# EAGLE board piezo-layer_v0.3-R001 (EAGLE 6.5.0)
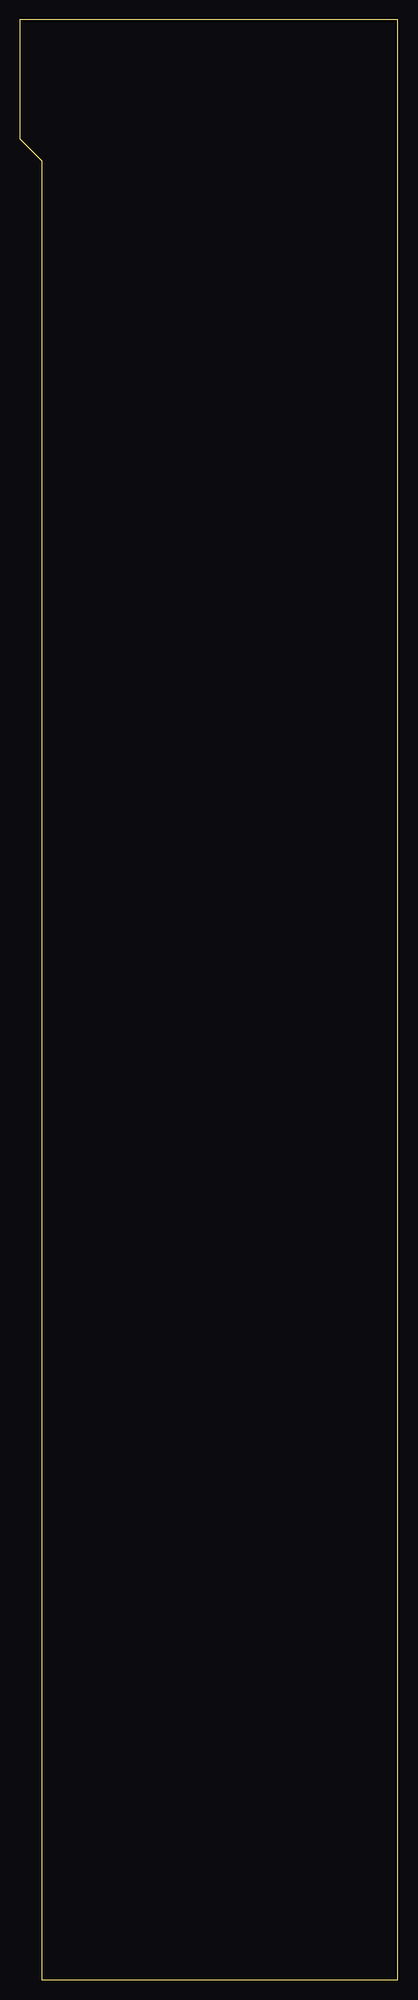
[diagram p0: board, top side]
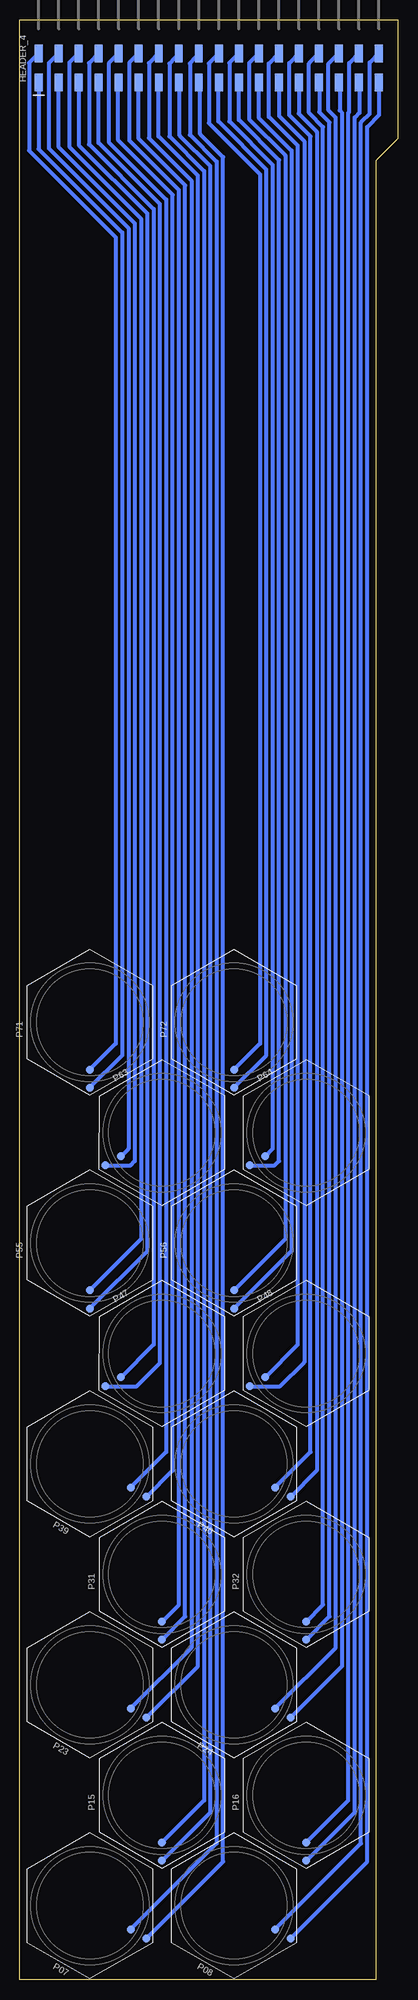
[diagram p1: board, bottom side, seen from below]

Size 48 x 248.5 mm. Coordinates in mm from the lower left corner, seen from the top.
Outline: 2.8,0 48,0 48,248.5 0,248.5 0,233.4 2.8,230.6 2.8,0
Copper layers (1*16): Top 0.009mm / dielectric 0.2mm / Bottom 0.018mm
Design rules "1L-0.2-0.15_0.3mm *": minimum track width 0.2mm, minimum drill 0.3mm, track to track 0.15mm, track to pad 0.15mm, pad to pad 0.15mm, via to via 0.15mm, smd to smd 0.15mm, copper to edge 0.5mm, drill to drill 1mm, minimum pad ring 10mil, minimum via ring 8mil, stop-mask expansion 4mil, vias tented up to drill 0mil, thermal gap 10mil

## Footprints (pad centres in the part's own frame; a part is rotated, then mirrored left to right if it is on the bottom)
2X18_2.54_90_SMD = smd 1 x 2.2: 1 -21.59,-1.84; 2 -21.59,1.84; 3 -19.05,-1.84; 4 -19.05,1.84; 5 -16.51,-1.84; 6 -16.51,1.84; 7 -13.97,-1.84; 8 -13.97,1.84; 9 -11.43,-1.84; 10 -11.43,1.84; 11 -8.89,-1.84; 12 -8.89,1.84; 13 -6.35,-1.84; 14 -6.35,1.84; 15 -3.81,-1.84; 16 -3.81,1.84; 17 -1.27,-1.84; 18 -1.27,1.84; 19 1.27,-1.84; 20 1.27,1.84; 21 3.81,-1.84; 22 3.81,1.84; 23 6.35,-1.84; 24 6.35,1.84; 25 8.89,-1.84; 26 8.89,1.84; 27 11.43,-1.84; 28 11.43,1.84; 29 13.97,-1.84; 30 13.97,1.84; 31 16.51,-1.84; 32 16.51,1.84; 33 19.05,-1.84; 34 19.05,1.84; 35 21.59,-1.84; 36 21.59,1.84
PIEZO-BENDER-HEX_16MM_1+_1- = smd 1 x 1: PAD1 -8.3,0; TIP1 -6,0

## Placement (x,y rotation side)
HEADER_4  HEADER_2X18-2.54_90_SMD  [2X18_2.54_90_SMD]  24,242.4 0 bottom
P07  PIEZO-BENDER-HEX_1-1  [PIEZO-BENDER-HEX_16MM_1+_1-]  39.1,9.4 150 bottom
P08  PIEZO-BENDER-HEX_1-1  [PIEZO-BENDER-HEX_16MM_1+_1-]  20.8,9.4 150 bottom
P15  PIEZO-BENDER-HEX_1-1  [PIEZO-BENDER-HEX_16MM_1+_1-]  29.95,23.4 90 bottom
P16  PIEZO-BENDER-HEX_1-1  [PIEZO-BENDER-HEX_16MM_1+_1-]  11.65,23.4 90 bottom
P23  PIEZO-BENDER-HEX_1-1  [PIEZO-BENDER-HEX_16MM_1+_1-]  39.1,37.4 150 bottom
P24  PIEZO-BENDER-HEX_1-1  [PIEZO-BENDER-HEX_16MM_1+_1-]  20.8,37.4 150 bottom
P31  PIEZO-BENDER-HEX_1-1  [PIEZO-BENDER-HEX_16MM_1+_1-]  29.95,51.4 90 bottom
P32  PIEZO-BENDER-HEX_1-1  [PIEZO-BENDER-HEX_16MM_1+_1-]  11.65,51.4 90 bottom
P39  PIEZO-BENDER-HEX_1-1  [PIEZO-BENDER-HEX_16MM_1+_1-]  39.1,65.4 150 bottom
P40  PIEZO-BENDER-HEX_1-1  [PIEZO-BENDER-HEX_16MM_1+_1-]  20.8,65.4 150 bottom
P47  PIEZO-BENDER-HEX_1-1  [PIEZO-BENDER-HEX_16MM_1+_1-]  29.95,79.4 30 bottom
P48  PIEZO-BENDER-HEX_1-1  [PIEZO-BENDER-HEX_16MM_1+_1-]  11.65,79.4 30 bottom
P55  PIEZO-BENDER-HEX_1-1  [PIEZO-BENDER-HEX_16MM_1+_1-]  39.1,93.4 90 bottom
P56  PIEZO-BENDER-HEX_1-1  [PIEZO-BENDER-HEX_16MM_1+_1-]  20.8,93.4 90 bottom
P63  PIEZO-BENDER-HEX_1-1  [PIEZO-BENDER-HEX_16MM_1+_1-]  29.95,107.4 30 bottom
P64  PIEZO-BENDER-HEX_1-1  [PIEZO-BENDER-HEX_16MM_1+_1-]  11.65,107.4 30 bottom
P71  PIEZO-BENDER-HEX_1-1  [PIEZO-BENDER-HEX_16MM_1+_1-]  39.1,121.4 90 bottom
P72  PIEZO-BENDER-HEX_1-1  [PIEZO-BENDER-HEX_16MM_1+_1-]  20.8,121.4 90 bottom

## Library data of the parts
HEADER_4 = SABRe
P07 P08 P15 P16 P23 P24 P31 P32 P39 P40 P47 P48 P55 P56 P63 P64 P71 P72 = ICST

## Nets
BUS+7: HEADER_4.18 P07.TIP1
BUS+8: HEADER_4.36 P08.TIP1
BUS+15: HEADER_4.16 P15.TIP1
BUS+16: HEADER_4.34 P16.TIP1
BUS+23: HEADER_4.14 P23.TIP1
BUS+24: HEADER_4.32 P24.TIP1
BUS+31: HEADER_4.12 P31.TIP1
BUS+32: HEADER_4.30 P32.TIP1
BUS+39: HEADER_4.10 P39.TIP1
BUS+40: HEADER_4.28 P40.TIP1
BUS+47: HEADER_4.8 P47.TIP1
BUS+48: HEADER_4.26 P48.TIP1
BUS+55: HEADER_4.6 P55.TIP1
BUS+56: HEADER_4.24 P56.TIP1
BUS+63: HEADER_4.4 P63.TIP1
BUS+64: HEADER_4.22 P64.TIP1
BUS+71: HEADER_4.2 P71.TIP1
BUS+72: HEADER_4.20 P72.TIP1
BUS-7: HEADER_4.17 P07.PAD1
BUS-8: HEADER_4.35 P08.PAD1
BUS-15: HEADER_4.15 P15.PAD1
BUS-16: HEADER_4.33 P16.PAD1
BUS-23: HEADER_4.13 P23.PAD1
BUS-24: HEADER_4.31 P24.PAD1
BUS-31: HEADER_4.11 P31.PAD1
BUS-32: HEADER_4.29 P32.PAD1
BUS-39: HEADER_4.9 P39.PAD1
BUS-40: HEADER_4.27 P40.PAD1
BUS-47: HEADER_4.7 P47.PAD1
BUS-48: HEADER_4.25 P48.PAD1
BUS-55: HEADER_4.5 P55.PAD1
BUS-56: HEADER_4.23 P56.PAD1
BUS-63: HEADER_4.3 P63.PAD1
BUS-64: HEADER_4.21 P64.PAD1
BUS-71: HEADER_4.1 P71.PAD1
BUS-72: HEADER_4.19 P72.PAD1

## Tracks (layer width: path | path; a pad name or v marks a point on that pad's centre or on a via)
BUS+7
  Bottom 0.5: P07.TIP1 23,17.3 23,230.5 26.4,233.9 26.4,242.98 HEADER_4.18
BUS+8
  Bottom 0.5: P08.TIP1 4.7,17.3 4.7,235.5 3.6,236.6 3.6,243.05 HEADER_4.36
BUS+15
  Bottom 0.5: P15.TIP1 24.6,22.75 24.6,229.3 29,233.7 29,242.92 HEADER_4.16
BUS+16
  Bottom 0.5: P16.TIP1 6.3,22.75 6.3,236.7 6.2,236.8 6.2,242.99 HEADER_4.34
BUS+23
  Bottom 0.5: P23.TIP1 26.2,42.1 26.2,228.1 31.6,233.5 31.6,242.99 HEADER_4.14
BUS+24
  Bottom 0.5: P24.TIP1 7.9,42.1 7.9,236.1 8.8,237 8.8,242.93 HEADER_4.32
BUS+31
  Bottom 0.5: P31.TIP1 27.8,47.55 27.8,226.9 34.1,233.2 34.1,243.03 HEADER_4.12
BUS+32
  Bottom 0.5: P32.TIP1 9.5,47.55 9.5,234.9 11.3,236.7 11.3,242.97 HEADER_4.30
BUS+39
  Bottom 0.5: P39.TIP1 29.4,66.9 29.4,225.7 36.7,233 36.7,242.97 HEADER_4.10
BUS+40
  Bottom 0.5: P40.TIP1 11.1,66.9 11.1,233.7 13.8,236.4 13.8,243.01 HEADER_4.28
BUS+47
  Bottom 0.5: P47.TIP1 31,80.55 31,224.5 39.2,232.7 39.2,243.01 HEADER_4.8
BUS+48
  Bottom 0.5: P48.TIP1 12.7,80.55 12.7,232.5 16.4,236.2 16.4,242.95 HEADER_4.26
BUS+55
  Bottom 0.5: P55.TIP1 32.6,93.9 32.6,223.3 41.7,232.4 41.7,243.05 HEADER_4.6
BUS+56
  Bottom 0.5: P56.TIP1 14.3,93.9 14.3,231.3 18.9,235.9 18.9,242.99 HEADER_4.24
BUS+63
  Bottom 0.5: P63.TIP1 34.2,105.35 34.2,222.1 44.3,232.2 44.3,242.99 HEADER_4.4
BUS+64
  Bottom 0.5: P64.TIP1 15.9,105.35 15.9,230.1 21.4,235.6 21.4,243.03 HEADER_4.22
BUS+71
  Bottom 0.5: P71.TIP1 35.8,118.7 35.8,220.9 46.8,231.9 46.8,243.03 HEADER_4.2
BUS+72
  Bottom 0.5: P72.TIP1 17.5,118.7 17.5,228.9 24,235.4 24,242.97 HEADER_4.20
BUS-7
  Bottom 0.5: P07.PAD1 22.2,14.96 22.2,231.1 25.1,234 25.1,240.52 HEADER_4.17
BUS-8
  Bottom 0.5: P08.PAD1 3.9,14.96 3.9,234.9 2.4,236.4 HEADER_4.35
BUS-15
  Bottom 0.5: P15.PAD1 23.8,21.25 23.8,229.9 27.7,233.8 27.7,240.54 HEADER_4.15
BUS-16
  Bottom 0.5: P16.PAD1 5.5,21.25 5.5,236.1 4.9,236.7 4.9,240.51 HEADER_4.33
BUS-23
  Bottom 0.5: P23.PAD1 25.4,39.76 25.4,228.7 30.4,233.7 30.4,240.51 HEADER_4.13
BUS-24
  Bottom 0.5: P24.PAD1 7.1,39.76 7.1,236.7 7.4,237 7.4,240.47 HEADER_4.31
BUS-31
  Bottom 0.5: P31.PAD1 27,46.05 27,227.5 32.9,233.4 HEADER_4.11
BUS-32
  Bottom 0.5: P32.PAD1 8.7,46.05 8.7,235.5 10,236.8 10,240.53 HEADER_4.29
BUS-39
  Bottom 0.5: P39.PAD1 28.6,64.56 28.6,226.3 35.5,233.2 35.5,240.49 HEADER_4.9
BUS-40
  Bottom 0.5: P40.PAD1 10.3,64.56 10.3,234.3 12.6,236.6 12.6,240.53 HEADER_4.27
BUS-47
  Bottom 0.5: P47.PAD1 33.15,75.25 30.2,78.2 30.2,225.1 38,232.9 38,240.53 HEADER_4.7
BUS-48
  Bottom 0.5: P48.PAD1 14.95,75.25 11.9,78.3 11.9,233.1 15.1,236.3 HEADER_4.25
BUS-55
  Bottom 0.5: P55.PAD1 31.8,92.4 31.8,223.9 40.5,232.6 HEADER_4.5
BUS-56
  Bottom 0.5: P56.PAD1 13.5,92.4 13.5,231.9 17.7,236.1 17.7,240.51 HEADER_4.23
BUS-63
  Bottom 0.5: P63.PAD1 33.95,103.25 33.4,103.8 33.4,222.7 43.1,232.4 43.1,240.51 HEADER_4.3
BUS-64
  Bottom 0.5: P64.PAD1 15.65,103.25 15.1,103.8 15.1,230.7 20.2,235.8 HEADER_4.21
BUS-71
  Bottom 0.5: P71.PAD1 35,117.2 35,221.5 45.6,232.1 HEADER_4.1
BUS-72
  Bottom 0.5: P72.PAD1 16.7,117.2 16.7,229.5 22.8,235.6 22.8,240.49 HEADER_4.19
